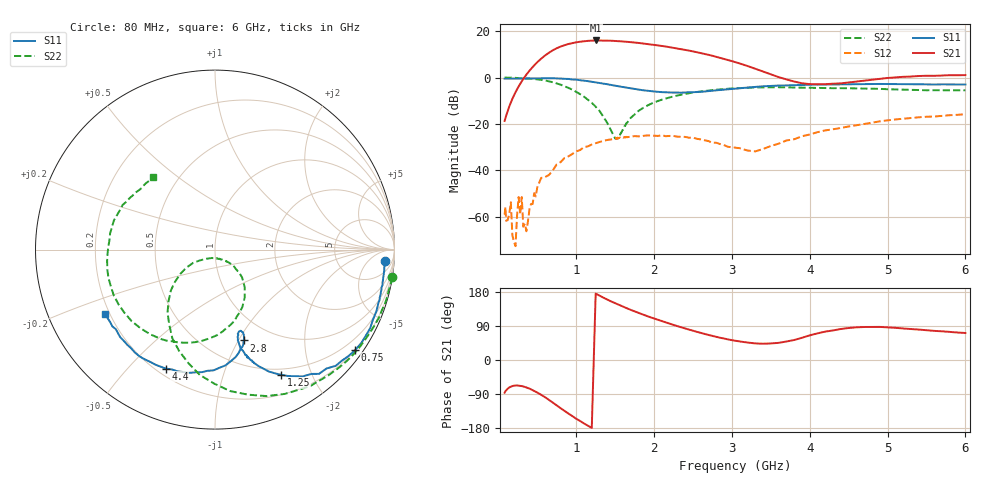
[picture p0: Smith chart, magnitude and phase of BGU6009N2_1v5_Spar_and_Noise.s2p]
! BGU6009N2, Vcc=1.5V, Icc= 5.0050 mA
# MHz S MA R 50
!  Freq-MHz  S11-mag  S11-arg  S21-mag  S21-arg  S12-mag  S12-arg  S22-mag  S22-arg
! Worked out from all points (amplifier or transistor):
!   130 points, 80 MHz to 6 GHz, reference 50 ohm
!   highest |S21| = 16.0 dB at 1.25 GHz (marker M1)
!   |S21| within 3 dB of that: 774.3 MHz to 2.219 GHz (1.445 GHz wide, 96.5 % of centre)
!   unconditionally stable (mu >= 1): start of sweep to 84.62 MHz; 97.02 MHz to 888.5 MHz; 1.133 GHz to end of sweep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
!   at 480 MHz: K = 1.76, MAG = 23.5 dB, |S12| = -51.2 dB
!   at 1.615 GHz: K = 1.09, MAG = 18.8 dB, |S12| = -25.8 dB
!   at 6 GHz: K = 1.43, MAG = 4.5 dB, |S12| = -15.8 dB
!   lowest NFmin = 0.79 dB at 1 GHz
!   S11 on the Smith chart (normalised r, x): 80 MHz: 15, -19; 750 MHz: 0.21, -3.10; 1.25 GHz: 0.42, -1.58; 2.8 GHz: 0.75, -1.05; 4.4 GHz: 0.23, -0.64; 6 GHz: 0.18, -0.27
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80  0.9496 -3.7  0.1166 -86.3  0.001116 -47.4  0.9962 -8.9
160  0.9503 -6.9  0.2909 -70.4  0.002063 138.8  0.994 -17.8
180  0.9498 -7.8  0.3498 -68.8  0.0004002 81.5  0.9892 -20.0
220  0.9501 -9.4  0.4834 -67.4  0.0002333 169.0  0.9855 -24.5
260  0.9515 -11.1  0.6425 -67.6  0.00267 154.9  0.9777 -29.0
360  0.9558 -15.4  1.159 -72.5  0.0004893 -170.8  0.9603 -40.6
480  0.9623 -20.8  1.978 -83.6  0.002745 162.7  0.9279 -55.0
600  0.9691 -26.8  2.992 -98.2  0.00719 -173.4  0.8655 -70.6
750  0.9611 -35.6  4.284 -120.0  0.01355 170.2  0.7474 -90.3
900  0.9336 -43.9  5.29 -141.3  0.02009 158.3  0.5991 -109.5
1100  0.8589 -55.3  6.051 -167.5  0.03184 137.3  0.3875 -131.9
1250  0.7904 -62.1  6.302 175.2  0.03856 123.1  0.236 -145.0
1510  0.6667 -70.9  6.143 148.9  0.04831 105.0  0.04762 -95.2
1640  0.6105 -73.8  5.928 137.4  0.05265 95.8  0.1001 -43.5
2100  0.4857 -74.9  4.799 102.4  0.05738 70.1  0.3338 -61.6
2450  0.4837 -71.8  3.809 80.2  0.05063 57.2  0.459 -84.8
2800  0.531 -72.5  2.799 61.1  0.03943 49.9  0.547 -108.5
3100  0.5906 -77.1  2.014 49.0  0.0301 61.7  0.5937 -127.2
4100  0.705 -104.5  0.7186 70.3  0.06668 107.3  0.5989 -178.0
4400  0.7176 -112.6  0.75 81.8  0.08205 104.6  0.5914 171.1
5100  0.7214 -130.4  1.006 85.0  0.1252 92.6  0.5553 148.8
6000  0.7093 -149.4  1.131 71.2  0.1625 77.4  0.5313 130.5
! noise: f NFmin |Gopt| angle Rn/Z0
1000  0.7855  0.3673  39.18  0.1801
1250  0.8377  0.3834  46.39  0.1723
1505  0.8395  0.3573  53.79  0.1682
1535  0.86  0.3868  50.37  0.1748
1560  0.8582  0.3659  53.9  0.1759
1590  0.8399  0.3642  50.36  0.1777
1620  0.8459  0.3659  53.94  0.1693
1645  0.8417  0.3654  57.73  0.164
1900  0.8916  0.3484  59.75  0.1724
2200  0.9073  0.3176  66.31  0.1995
